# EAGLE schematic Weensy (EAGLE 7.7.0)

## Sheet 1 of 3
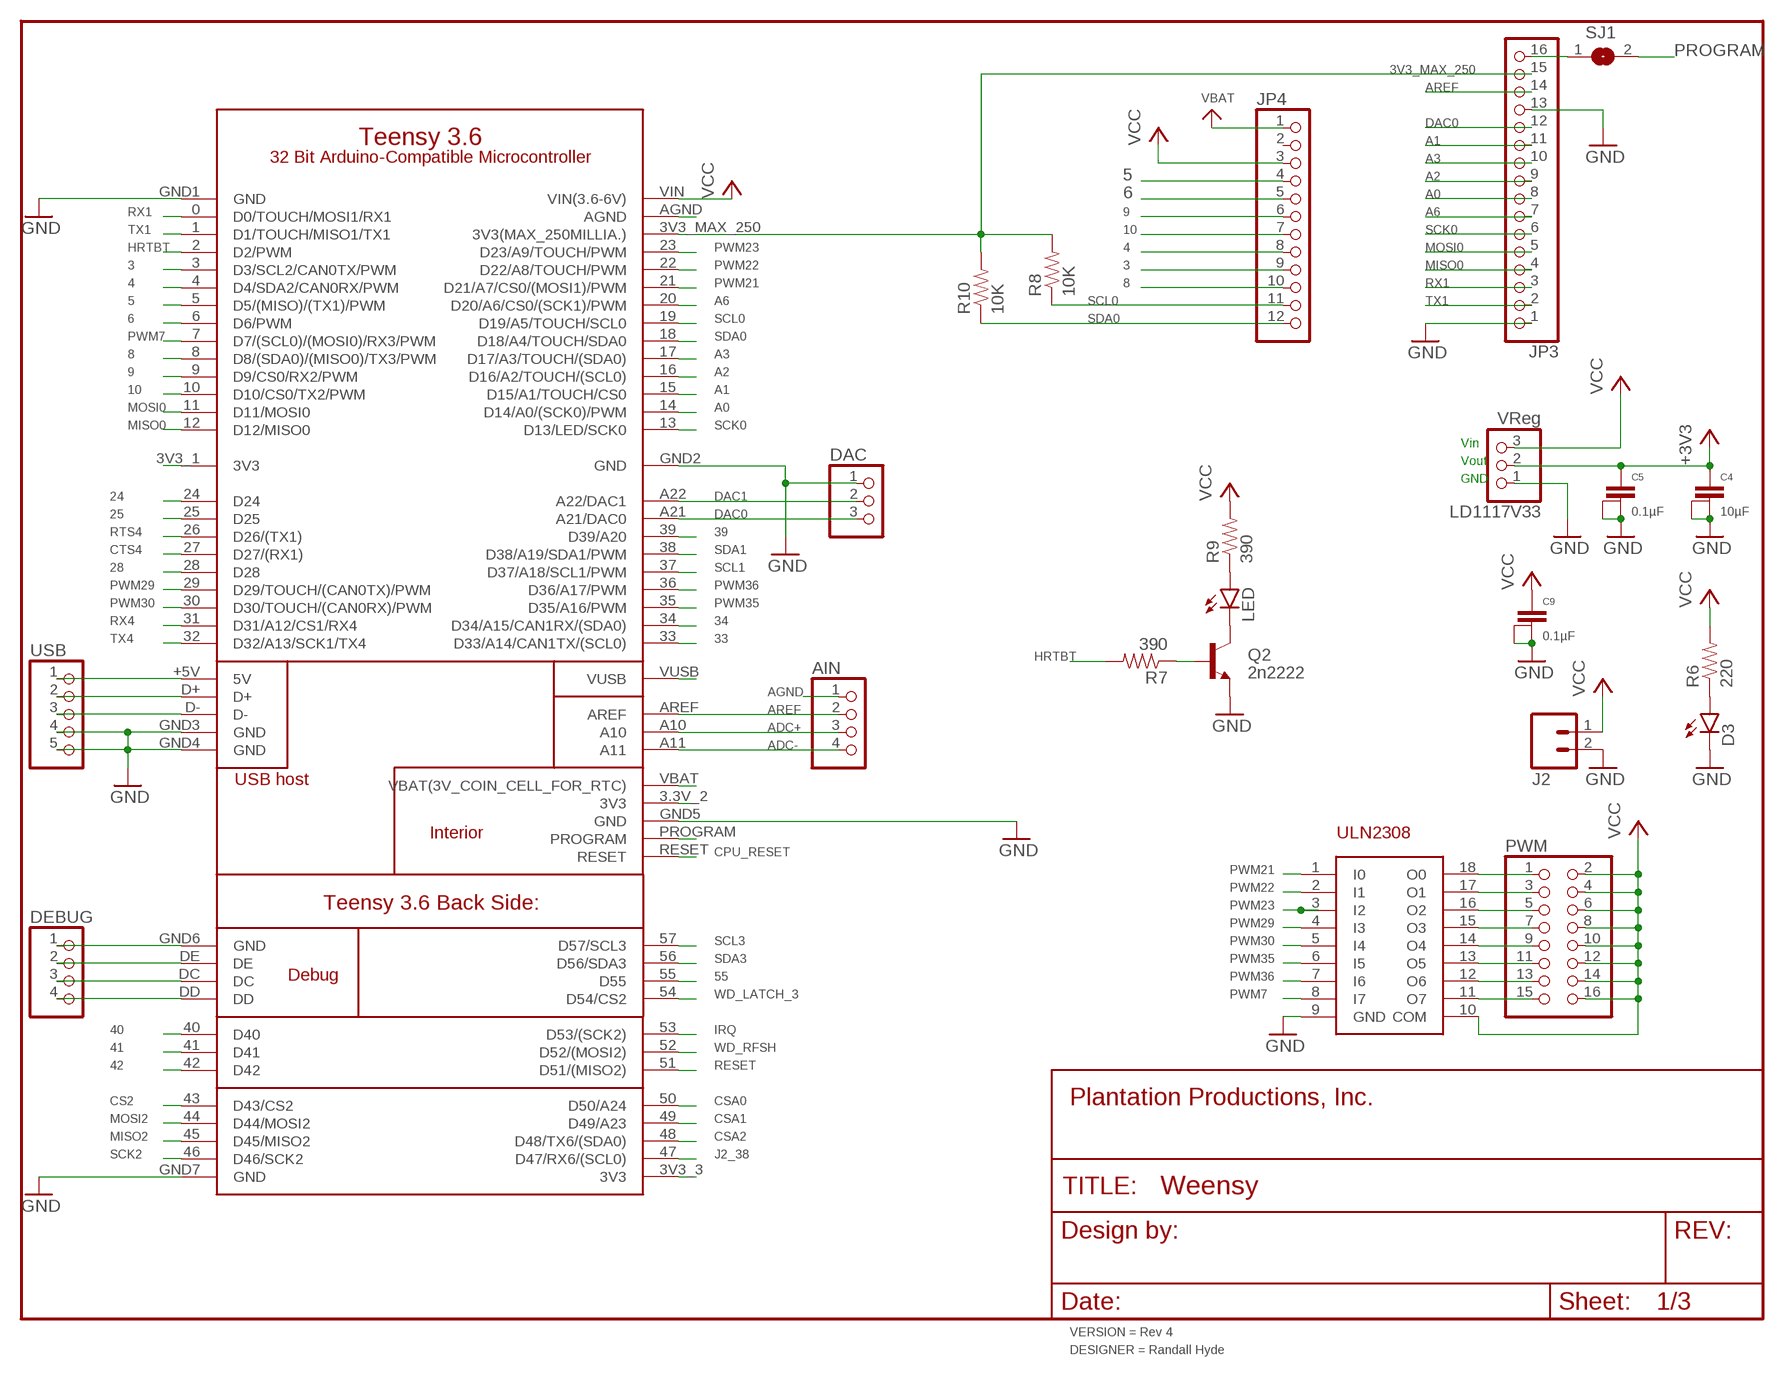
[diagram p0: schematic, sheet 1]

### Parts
AIN  PINHD-1X4  [1X04]
C4  10µF  CAPACITOR  [1+2CAP]
C5  0.1µF  CAPACITOR  [1+2CAP]
C9  0.1µF  CAPACITOR  [1+2CAP]
D3  LED5MM  [LED5MM]
DAC  PINHD-1X3  [1X03]
DEBUG  PINHD-1X4  [1X04]
FRAME1  FRAME-LETTERNO_PACKAGE  [DUMMY]
J2  M025MM  [SCREWTERMINAL-5MM-2]
JP3  HEADER-1X16ROUND  [1X16_ROUND]
JP4  HEADER-1X12  [1X12_ROUND]
LD1117V33  VReg  PINHD-1X3  [1X03]
LED  LED5MM  [LED5MM]
PWM  PINHD-2X8  [2X08]
Q2  2n2222  TRANSISTOR_NPNP2N2222A  [TO-92]
R6  220  1KOHM-1/4W-1%(PTH)  [AXIAL-0.3]
R7  390  10KOHM-1/4W-1%(PTH)HORIZ  [AXIAL-0.3]
R8  10K  10KOHM-1/4W-1%(PTH)HORIZ  [AXIAL-0.3]
R9  390  10KOHM-1/4W-1%(PTH)HORIZ  [AXIAL-0.3]
R10  10K  10KOHM-1/4W-1%(PTH)HORIZ  [AXIAL-0.3]
SJ1  SOLDERJUMPERCLOSED  [SOLDERJUMPER_CLOSEDWIRE]
U$1  TEENSY-3.6_FULL  [TEENSY-3.6_FULL]
ULN2308  ULN2308  [DIL18]
USB  PINHD-1X5  [1X05]

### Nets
3: JP4.9 U$1.3(D3/SCL2/CAN0TX/PWM)
3V3_MAX_250: JP3.15 R8.P$2 R10.P$2 U$1.3V3_MAX_250(3V3(MAX_250MILLIA.))
4: JP4.8 U$1.4(D4/SDA2/CAN0RX/PWM)
5: JP4.4 U$1.5(D5/(MISO)/(TX1)/PWM)
6: JP4.5 U$1.6(D6/PWM)
8: JP4.10 U$1.8(D8/(SDA0)/(MISO0)/TX3/PWM)
9: JP4.6 U$1.9(D9/CS0/RX2/PWM)
10: JP4.7 U$1.10(D10/CS0/TX2/PWM)
24: U$1.24(D24) ; also sheet 2
25: U$1.25(D25) ; also sheet 2
28: U$1.28(D28) ; also sheet 2
33: U$1.33(D33/A14/CAN1TX/(SCL0)) ; also sheet 2
34: U$1.34(D34/A15/CAN1RX/(SDA0)) ; also sheet 2
39: U$1.39(D39/A20) ; also sheet 2
40: U$1.40(D40) ; also sheet 2
41: U$1.41(D41) ; also sheet 2
42: U$1.42(D42) ; also sheet 2
55: U$1.55(D55) ; also sheet 2
+3V3 [Power]: C4.1 C5.1 LD1117V33.2 ; also sheet 2,3
A0: JP3.8 U$1.14(D14/A0/(SCK0)/PWM)
A1: JP3.11 U$1.15(D15/A1/TOUCH/CS0)
A2: JP3.9 U$1.16(D16/A2/TOUCH/(SCL0))
A3: JP3.10 U$1.17(D17/A3/TOUCH/(SDA0))
A6: JP3.7 U$1.20(D20/A6/CS0/(SCK1)/PWM)
ADC+: AIN.3 U$1.A10
ADC-: AIN.4 U$1.A11
AGND: AIN.1 U$1.AGND
AREF: AIN.2 JP3.14 U$1.AREF
CPU_RESET: U$1.RESET
CS2: U$1.43(D43/CS2) ; also sheet 3
CSA0: U$1.50(D50/A24) ; also sheet 3
CSA1: U$1.49(D49/A23) ; also sheet 3
CSA2: U$1.48(D48/TX6/(SDA0)) ; also sheet 3
CTS4: U$1.27(D27/(RX1)) ; also sheet 3
DAC0: DAC.3 JP3.12 U$1.A21(A21/DAC0)
DAC1: DAC.2 U$1.A22(A22/DAC1)
GND: C4.2@1 C4.2@2 C5.2@1 C5.2@2 C9.2@1 C9.2@2 D3.K(C) DAC.1 DEBUG.1 J2.2 JP3.1 JP3.13 LD1117V33.1 Q2.3(E) U$1.GND1(GND) U$1.GND2(GND) U$1.GND3(GND) U$1.GND4(GND) U$1.GND5(GND) U$1.GND6(GND) U$1.GND7(GND) ULN2308.9(GND) USB.4 USB.5 ; also sheet 2,3
HRTBT: R7.P$2 U$1.2(D2/PWM)
IRQ: U$1.53(D53/(SCK2)) ; also sheet 2
J2_38: U$1.47(D47/RX6/(SCL0)) ; also sheet 2
MISO0: JP3.4 U$1.12(D12/MISO0)
MISO2: U$1.45(D45/MISO2) ; also sheet 2
MOSI0: JP3.5 U$1.11(D11/MOSI0)
MOSI2: U$1.44(D44/MOSI2) ; also sheet 2
N$2: D3.A R6.P$1
N$20 [Power]: U$1.3V3_3(3V3)
N$23 [Hi Current]: PWM.1 ULN2308.18(O0)
N$24 [Hi Current]: PWM.3 ULN2308.17(O1)
N$25 [Hi Current]: PWM.5 ULN2308.16(O2)
N$26 [Hi Current]: PWM.7 ULN2308.15(O3)
N$27 [Hi Current]: PWM.9 ULN2308.14(O4)
N$28 [Hi Current]: PWM.11 ULN2308.13(O5)
N$29 [Hi Current]: PWM.13 ULN2308.12(O6)
N$30 [Hi Current]: PWM.15 ULN2308.11(O7)
N$31: U$1.3V3_1(3V3)
N$36: LED.K(C) Q2.1(C)
N$37: Q2.2(B) R7.P$1
N$38: LED.A R9.P$1
N$41: U$1.+5V(5V) USB.1
N$42: U$1.D+ USB.2
N$43: U$1.D- USB.3
N$46: DEBUG.2 U$1.DE
N$47: DEBUG.3 U$1.DC
N$48: DEBUG.4 U$1.DD
N$71: U$1.3.3V_2(3V3)
PROGRAM: SJ1.2 U$1.PROGRAM
PWM7: U$1.7(D7/(SCL0)/(MOSI0)/RX3/PWM) ULN2308.8(I7)
PWM21: U$1.21(D21/A7/CS0/(MOSI1)/PWM) ULN2308.1(I0)
PWM22: U$1.22(D22/A8/TOUCH/PWM) ULN2308.2(I1)
PWM23: U$1.23(D23/A9/TOUCH/PWM) ULN2308.3(I2)
PWM29: U$1.29(D29/TOUCH/(CAN0TX)/PWM) ULN2308.4(I3)
PWM30: U$1.30(D30/TOUCH/(CAN0RX)/PWM) ULN2308.5(I4)
PWM35: U$1.35(D35/A16/PWM) ULN2308.6(I5)
PWM36: U$1.36(D36/A17/PWM) ULN2308.7(I6)
RESET: U$1.51(D51/(MISO2)) ; also sheet 2,3
RST/BOOT: JP3.16 SJ1.1
RTS4: U$1.26(D26/(TX1)) ; also sheet 3
RX1: JP3.3 U$1.0(D0/TOUCH/MOSI1/RX1)
RX4: U$1.31(D31/A12/CS1/RX4) ; also sheet 3
SCK0: JP3.6 U$1.13(D13/LED/SCK0)
SCK2: U$1.46(D46/SCK2) ; also sheet 2,3
SCL0: JP4.11 R8.P$1 U$1.19(D19/A5/TOUCH/SCL0)
SCL1: U$1.37(D37/A18/SCL1/PWM) ; also sheet 2
SCL3: U$1.57(D57/SCL3) ; also sheet 2
SDA0: JP4.12 R10.P$1 U$1.18(D18/A4/TOUCH/SDA0)
SDA1: U$1.38(D38/A19/SDA1/PWM) ; also sheet 2
SDA3: U$1.56(D56/SDA3) ; also sheet 2
TX1: JP3.2 U$1.1(D1/TOUCH/MISO1/TX1)
TX4: U$1.32(D32/A13/SCK1/TX4) ; also sheet 3
VBAT: JP4.1 U$1.VBAT(VBAT(3V_COIN_CELL_FOR_RTC))
VCC [Hi Current]: C9.1 J2.1 JP4.3 LD1117V33.3 PWM.2 PWM.4 PWM.6 PWM.8 PWM.10 PWM.12 PWM.14 PWM.16 R6.P$2 R9.P$2 U$1.VIN(VIN(3.6-6V)) ULN2308.10(COM) ; also sheet 2,3
VUSB: U$1.VUSB
WD_LATCH_3: U$1.54(D54/CS2) ; also sheet 2
WD_RFSH: U$1.52(D52/(MOSI2)) ; also sheet 2
Unconnected: JP4.2

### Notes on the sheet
- Vin
- Vout
- GND

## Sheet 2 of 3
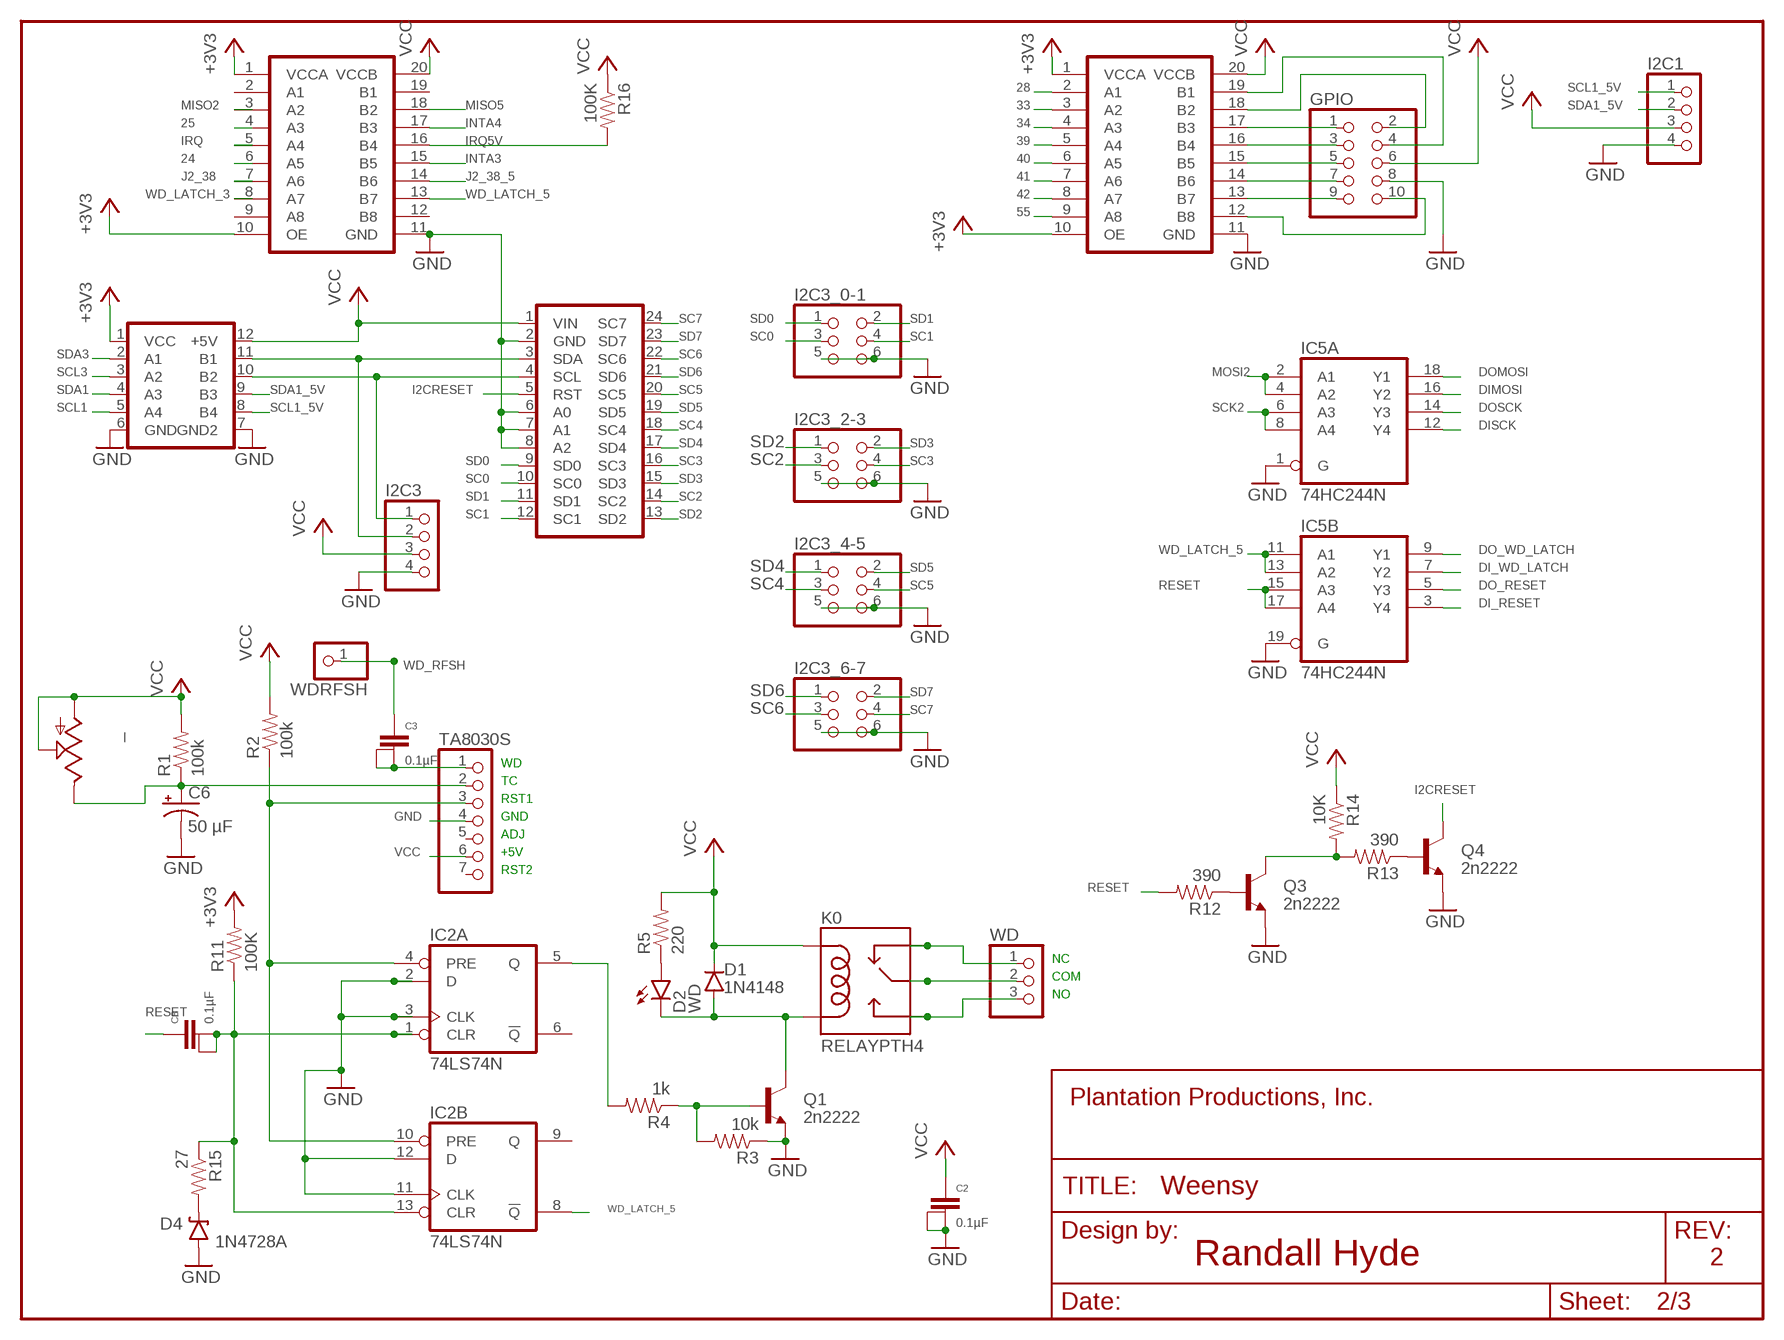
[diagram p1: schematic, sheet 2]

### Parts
_  TRIM_US-B64Y  [B64Y]
BOB1  ADAFRTTXB0108  [DIL20W]
BOB2  ADAFRTBSS138  [DIL12W]
BOB3  ADAFRTTCA9584  [DIL24W]
BOB4  ADAFRTTXB0108  [DIL20W]
C2  0.1µF  CAPACITOR  [1+2CAP]
C3  0.1µF  CAPACITOR  [1+2CAP]
C6  50 µF  100UF-25V-20%(PTH)  [CPOL-RADIAL-100UF-25V]
C8  0.1µF  CAPACITOR  [1+2CAP]
D1  1N4148  DIODE1N4148  [DIODE-1N4148]
D2  WD  LED5MM  [LED5MM]
D4  1N4728A  DIODE-ZENERPTH  [DIODE-ZENER]
FRAME2  FRAME-LETTERNO_PACKAGE  [DUMMY]
GPIO  PINHD-2X5  [2X05]
I2C1  PINHD-1X4  [1X04]
I2C3  PINHD-1X4  [1X04]
I2C3_0-1  PINHD-2X3  [2X03]
I2C3_2-3  PINHD-2X3  [2X03]
I2C3_4-5  PINHD-2X3  [2X03]
I2C3_6-7  PINHD-2X3  [2X03]
IC2  74LS74N  [DIL14]
IC5  74HC244N  [DIL20]
K0  RELAYPTH4  [RELAY-JZC]
Q1  2n2222  TRANSISTOR_NPNP2N2222A  [TO-92]
Q3  2n2222  TRANSISTOR_NPNP2N2222A  [TO-92]
Q4  2n2222  TRANSISTOR_NPNP2N2222A  [TO-92]
R1  100k  10KOHM-1/4W-1%(PTH)HORIZ  [AXIAL-0.3]
R2  100k  10KOHM-1/4W-1%(PTH)HORIZ  [AXIAL-0.3]
R3  10k  10KOHM-1/4W-1%(PTH)HORIZ  [AXIAL-0.3]
R4  1k  10KOHM-1/4W-1%(PTH)HORIZ  [AXIAL-0.3]
R5  220  10KOHM-1/4W-1%(PTH)HORIZ  [AXIAL-0.3]
R11  100K  1KOHM-1/4W-1%(PTH)  [AXIAL-0.3]
R12  390  10KOHM-1/4W-1%(PTH)HORIZ  [AXIAL-0.3]
R13  390  10KOHM-1/4W-1%(PTH)HORIZ  [AXIAL-0.3]
R14  10K  10KOHM-1/4W-1%(PTH)HORIZ  [AXIAL-0.3]
R15  27  1KOHM-1/4W-1%(PTH)  [AXIAL-0.3]
R16  100K  10KOHM-1/4W-1%(PTH)HORIZ  [AXIAL-0.3]
TA8030S  PINHD-1X7  [1X07]
WD  PINHD-1X3  [1X03]
WDRFSH  PINHD-1X1  [1X01]

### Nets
24: BOB1.6(A5) ; also sheet 1
25: BOB1.4(A3) ; also sheet 1
28: BOB4.2(A1) ; also sheet 1
33: BOB4.3(A2) ; also sheet 1
34: BOB4.4(A3) ; also sheet 1
39: BOB4.5(A4) ; also sheet 1
40: BOB4.6(A5) ; also sheet 1
41: BOB4.7(A6) ; also sheet 1
42: BOB4.8(A7) ; also sheet 1
55: BOB4.9(A8) ; also sheet 1
+3V3 [Power]: BOB1.1(VCCA) BOB1.10(OE) BOB2.1(VCC) BOB4.1(VCCA) BOB4.10(OE) R11.P$2 ; also sheet 1,3
DI_RESET: IC5.3(B:Y4) ; also sheet 3
DI_WD_LATCH: IC5.7(B:Y2) ; also sheet 3
DIMOSI: IC5.16(A:Y2) ; also sheet 3
DISCK: IC5.12(A:Y4) ; also sheet 3
DO_RESET: IC5.5(B:Y3) ; also sheet 3
DO_WD_LATCH: IC5.9(B:Y1) ; also sheet 3
DOMOSI: IC5.18(A:Y1) ; also sheet 3
DOSCK: IC5.14(A:Y3) ; also sheet 3
GND: BOB1.11(GND) BOB2.6(GND) BOB2.7(GND2) BOB3.2(GND) BOB3.6(A0) BOB3.7(A1) BOB3.8(A2) BOB4.11(GND) C2.2@1 C2.2@2 C6.2(-) D4.P$2(A) GPIO.8 I2C1.4 I2C3.4 I2C3_0-1.5 I2C3_0-1.6 I2C3_2-3.5 I2C3_2-3.6 I2C3_4-5.5 I2C3_4-5.6 I2C3_6-7.5 I2C3_6-7.6 IC2.2(A:D) IC2.3(A:CLK) IC2.11(B:CLK) IC2.12(B:D) IC5.1(A:G) IC5.19(B:G) Q1.3(E) Q3.3(E) Q4.3(E) R3.P$1 TA8030S.4 ; also sheet 1,3
GPIO28: BOB4.19(B1) GPIO.4
GPIO33: BOB4.18(B2) GPIO.2
GPIO34: BOB4.17(B3) GPIO.1
GPIO39: BOB4.16(B4) GPIO.3
GPIO40: BOB4.15(B5) GPIO.5
GPIO41: BOB4.14(B6) GPIO.7
GPIO42: BOB4.13(B7) GPIO.9
GPIO55: BOB4.12(B8) GPIO.10
I2CRESET: BOB3.5(RST) Q4.1(C)
INTA3: BOB1.15(B5) ; also sheet 3
INTA4: BOB1.17(B3) ; also sheet 3
IRQ: BOB1.5(A4) ; also sheet 1
IRQ5V: BOB1.16(B4) R16.P$2 ; also sheet 3
J2_38: BOB1.7(A6) ; also sheet 1
J2_38_5: BOB1.14(B6) ; also sheet 3
MISO2: BOB1.3(A2) ; also sheet 1
MISO5: BOB1.18(B2) ; also sheet 3
MOSI2: IC5.2(A:A1) IC5.4(A:A2) ; also sheet 1
N$3: C3.2@1 C3.2@2 TA8030S.1
N$4: _.E C6.1(+) R1.P$1 TA8030S.2
N$5: BOB2.11(B1) BOB3.3(SDA) I2C3.2
N$6: D1.A D2.K(C) K0.1(COIL2) Q1.1(C)
N$9: D2.A R5.P$1
N$11: Q1.2(B) R3.P$2 R4.P$1
N$12: Q3.2(B) R12.P$1
N$13: Q4.2(B) R13.P$1
N$14 [Power]: K0.4(MAIN) WD.2
N$15 [Power]: K0.3(NO) WD.3
N$16: BOB2.10(B2) BOB3.4(SCL) I2C3.1
N$17: Q3.1(C) R13.P$2 R14.P$2
N$39: D4.P$1(C) R15.P$2
NC [Power]: K0.2(NC) WD.1
RESET: C8.1 IC5.15(B:A3) IC5.17(B:A4) R12.P$2 ; also sheet 1,3
RESETWD: C8.2@1 C8.2@2 IC2.1(A:CLR) IC2.13(B:CLR) R11.P$1 R15.P$1
RST1: IC2.4(A:PRE) IC2.10(B:PRE) R2.P$1 TA8030S.3
SC0: BOB3.10(SC0) I2C3_0-1.3
SC1: BOB3.12(SC1) I2C3_0-1.4
SC2: BOB3.14(SC2) I2C3_2-3.3
SC3: BOB3.16(SC3) I2C3_2-3.4
SC4: BOB3.18(SC4) I2C3_4-5.3
SC5: BOB3.20(SC5) I2C3_4-5.4
SC6: BOB3.22(SC6) I2C3_6-7.3
SC7: BOB3.24(SC7) I2C3_6-7.4
SCK2: IC5.6(A:A3) IC5.8(A:A4) ; also sheet 1,3
SCL1: BOB2.5(A4) ; also sheet 1
SCL1_5V: BOB2.8(B4) I2C1.1
SCL3: BOB2.3(A2) ; also sheet 1
SD0: BOB3.9(SD0) I2C3_0-1.1
SD1: BOB3.11(SD1) I2C3_0-1.2
SD2: BOB3.13(SD2) I2C3_2-3.1
SD3: BOB3.15(SD3) I2C3_2-3.2
SD4: BOB3.17(SD4) I2C3_4-5.1
SD5: BOB3.19(SD5) I2C3_4-5.2
SD6: BOB3.21(SD6) I2C3_6-7.1
SD7: BOB3.23(SD7) I2C3_6-7.2
SDA1: BOB2.4(A3) ; also sheet 1
SDA1_5V: BOB2.9(B3) I2C1.2
SDA3: BOB2.2(A1) ; also sheet 1
VCC [Hi Current]: _.A _.S BOB1.20(VCCB) BOB2.12(+5V) BOB3.1(VIN) BOB4.20(VCCB) C2.1 D1.C GPIO.6 I2C1.3 I2C3.3 K0.5(COIL1) R1.P$2 R2.P$2 R5.P$2 R14.P$1 R16.P$1 TA8030S.6 ; also sheet 1,3
WD_LATCH_3: BOB1.8(A7) ; also sheet 1
WD_LATCH_5: BOB1.13(B7) IC2.8(B:!Q) IC5.11(B:A1) IC5.13(B:A2)
WD_RFSH: C3.1 WDRFSH.1 ; also sheet 1
WDOUT: IC2.5(A:Q) R4.P$2
Unconnected: BOB1.2(A1) BOB1.9(A8) BOB1.12(B8) BOB1.19(B1) IC2.6(A:!Q) IC2.9(B:Q) TA8030S.5 TA8030S.7

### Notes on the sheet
- WD
- TC
- RST1
- GND
- ADJ
- +5V
- RST2
- NC
- COM
- NO
- Randall Hyde | 2

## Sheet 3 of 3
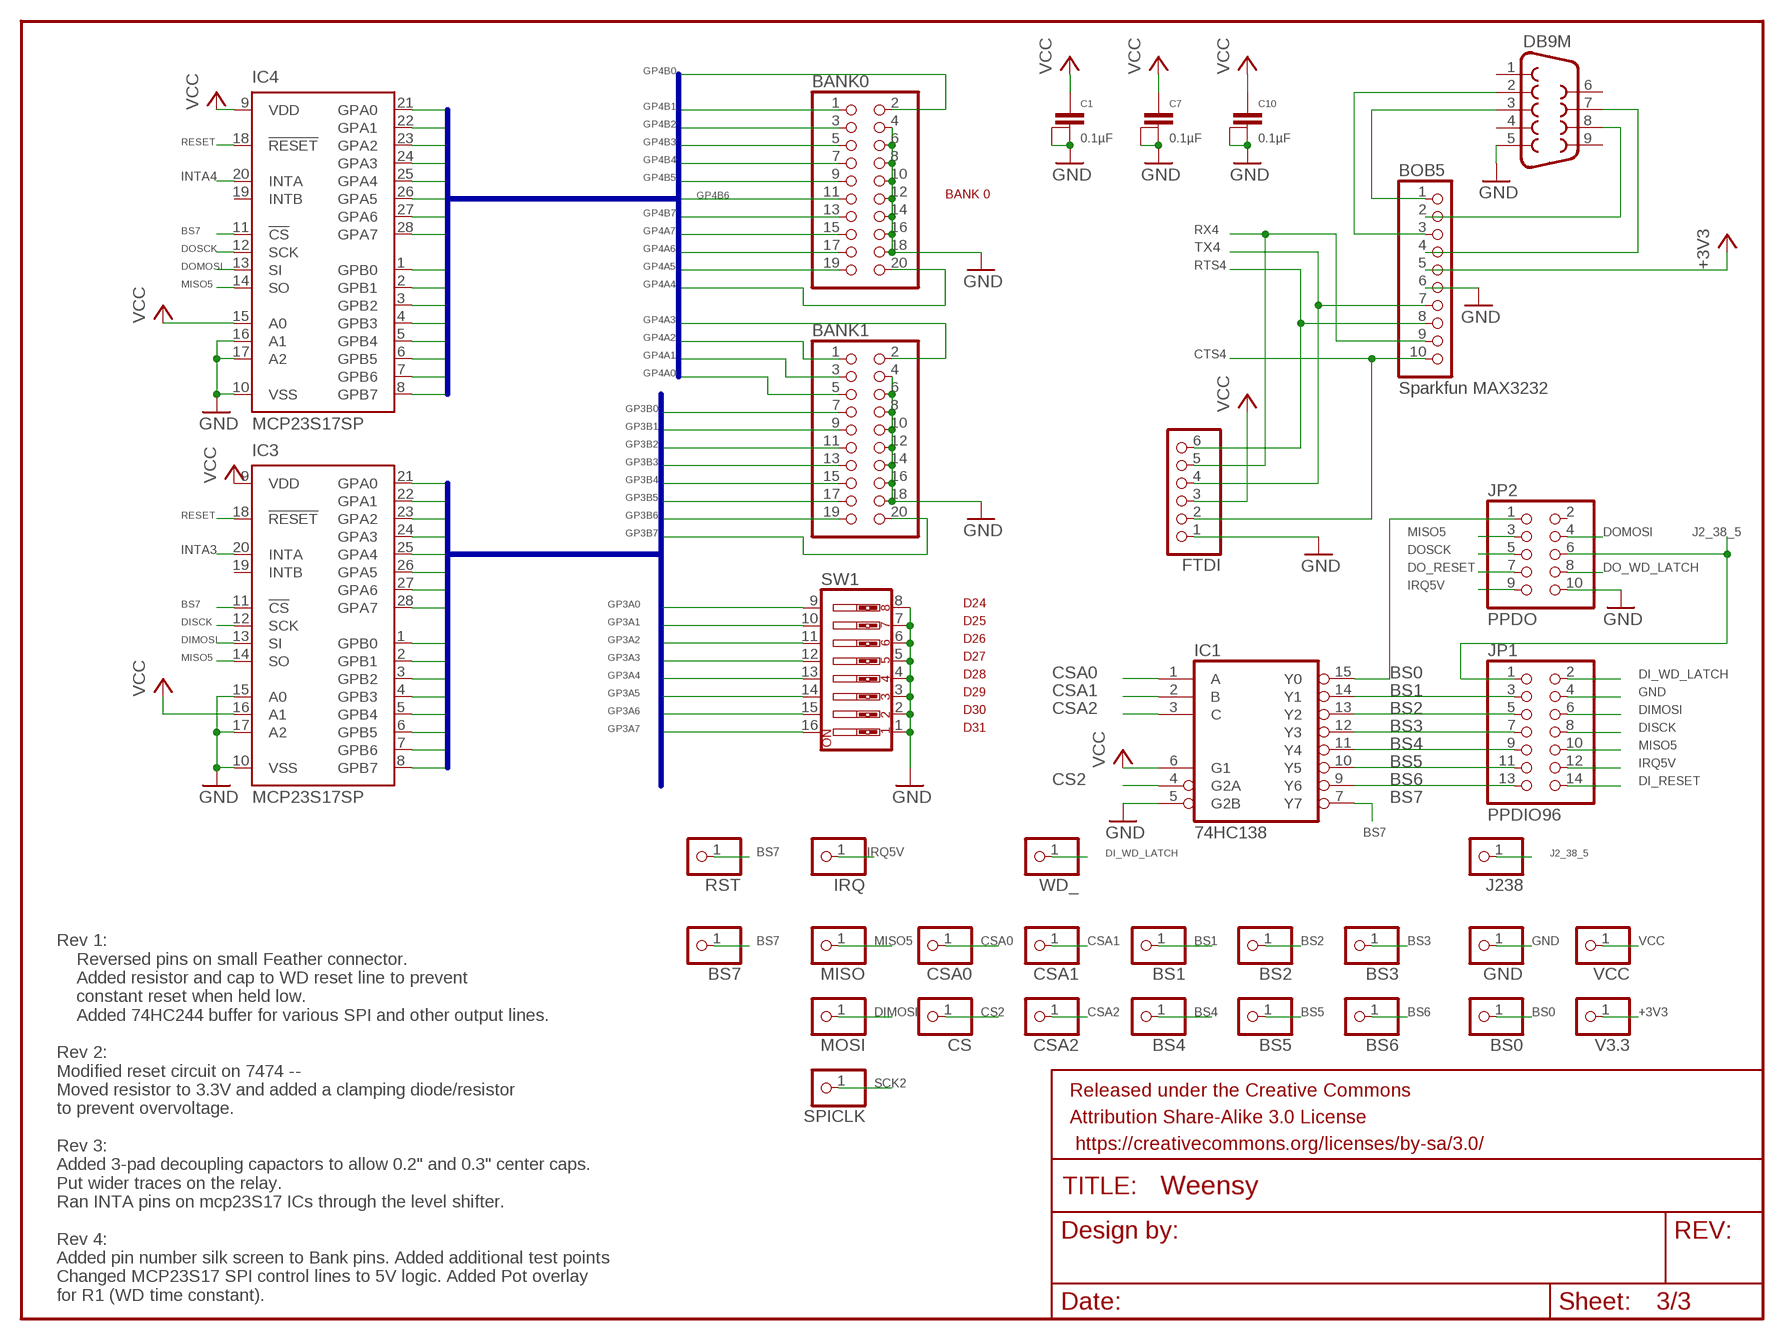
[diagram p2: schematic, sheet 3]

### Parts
BANK0  PINHD-2X10  [2X10]
BANK1  PINHD-2X10  [2X10]
BOB5  Sparkfun MAX3232  PINHD-1X10  [1X10]
BS0  PINHD-1X1  [1X01]
BS1  PINHD-1X1  [1X01]
BS2  PINHD-1X1  [1X01]
BS3  PINHD-1X1  [1X01]
BS4  PINHD-1X1  [1X01]
BS5  PINHD-1X1  [1X01]
BS6  PINHD-1X1  [1X01]
BS7  PINHD-1X1  [1X01]
C1  0.1µF  CAPACITOR  [1+2CAP]
C7  0.1µF  CAPACITOR  [1+2CAP]
C10  0.1µF  CAPACITOR  [1+2CAP]
CS  PINHD-1X1  [1X01]
CSA0  PINHD-1X1  [1X01]
CSA1  PINHD-1X1  [1X01]
CSA2  PINHD-1X1  [1X01]
DB9M  DB9MALE  [DB9_MALE]
FRAME3  FRAME-LETTER  [CREATIVE_COMMONS]
FTDI  PINHD-1X6  [1X06]
GND  PINHD-1X1  [1X01]
IC1  74HC138  74LS138N  [DIL16]
IC3  MCP23S17SP  [DIL28-3]
IC4  MCP23S17SP  [DIL28-3]
IRQ  PINHD-1X1  [1X01]
J238  PINHD-1X1  [1X01]
JP1  PPDIO96  PINHD-2X7  [2X07]
JP2  PPDO  PINHD-2X5  [2X05]
MISO  PINHD-1X1  [1X01]
MOSI  PINHD-1X1  [1X01]
RST  PINHD-1X1  [1X01]
SPICLK  PINHD-1X1  [1X01]
SW1  SW_DIP-8  [DIPSWITCH-08]
V3.3  PINHD-1X1  [1X01]
VCC  PINHD-1X1  [1X01]
WD_  PINHD-1X1  [1X01]

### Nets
+3V3 [Power]: BOB5.5 V3.3.1 ; also sheet 1,2
BS0: BS0.1 IC1.15(Y0) JP2.1
BS1: BS1.1 IC1.14(Y1) JP1.3
BS2: BS2.1 IC1.13(Y2) JP1.5
BS3: BS3.1 IC1.12(Y3) JP1.7
BS4: BS4.1 IC1.11(Y4) JP1.9
BS5: BS5.1 IC1.10(Y5) JP1.11
BS6: BS6.1 IC1.9(Y6) JP1.13
BS7: BS7.1 IC1.7(Y7) IC3.11(!CS) IC4.11(!CS) RST.1
CS2: CS.1 IC1.4(G2A) ; also sheet 1
CSA0: CSA0.1 IC1.1(A) ; also sheet 1
CSA1: CSA1.1 IC1.2(B) ; also sheet 1
CSA2: CSA2.1 IC1.3(C) ; also sheet 1
CTS4: BOB5.10 FTDI.2 ; also sheet 1
DI_RESET: JP1.14 ; also sheet 2
DI_WD_LATCH: JP1.2 WD_.1 ; also sheet 2
DIMOSI: IC3.13(SI) JP1.6 MOSI.1 ; also sheet 2
DISCK: IC3.12(SCK) JP1.8 ; also sheet 2
DO_RESET: JP2.7 ; also sheet 2
DO_WD_LATCH: JP2.8 ; also sheet 2
DOMOSI: IC4.13(SI) JP2.4 ; also sheet 2
DOSCK: IC4.12(SCK) JP2.5 ; also sheet 2
GND: BANK0.4 BANK0.6 BANK0.8 BANK0.10 BANK0.12 BANK0.14 BANK0.16 BANK0.18 BANK1.4 BANK1.6 BANK1.8 BANK1.10 BANK1.12 BANK1.14 BANK1.16 BANK1.18 BOB5.6 C1.2@1 C1.2@2 C7.2@1 C7.2@2 C10.2@1 C10.2@2 DB9M.5 FTDI.1 GND.1 IC1.5(G2B) IC3.10(VSS) IC3.15(A0) IC3.17(A2) IC4.10(VSS) IC4.16(A1) IC4.17(A2) JP1.4 JP2.10 SW1.1 SW1.2 SW1.3 SW1.4 SW1.5 SW1.6 SW1.7 SW1.8 ; also sheet 1,2
GP3A0: IC3.28(GPA7) SW1.9
GP3A1: IC3.27(GPA6) SW1.10
GP3A2: IC3.26(GPA5) SW1.11
GP3A3: IC3.25(GPA4) SW1.12
GP3A4: IC3.24(GPA3) SW1.13
GP3A5: IC3.23(GPA2) SW1.14
GP3A6: IC3.22(GPA1) SW1.15
GP3A7: IC3.21(GPA0) SW1.16
GP3B0: BANK1.7 IC3.1(GPB0)
GP3B1: BANK1.9 IC3.2(GPB1)
GP3B2: BANK1.11 IC3.3(GPB2)
GP3B3: BANK1.13 IC3.4(GPB3)
GP3B4: BANK1.15 IC3.5(GPB4)
GP3B5: BANK1.17 IC3.6(GPB5)
GP3B6: BANK1.19 IC3.7(GPB6)
GP3B7: BANK1.20 IC3.8(GPB7)
GP4A0: BANK1.5 IC4.21(GPA0)
GP4A1: BANK1.3 IC4.22(GPA1)
GP4A2: BANK1.1 IC4.23(GPA2)
GP4A3: BANK1.2 IC4.24(GPA3)
GP4A4: BANK0.20 IC4.25(GPA4)
GP4A5: BANK0.19 IC4.26(GPA5)
GP4A6: BANK0.17 IC4.27(GPA6)
GP4A7: BANK0.15 IC4.28(GPA7)
GP4B0: BANK0.2 IC4.1(GPB0)
GP4B1: BANK0.1 IC4.2(GPB1)
GP4B2: BANK0.3 IC4.3(GPB2)
GP4B3: BANK0.5 IC4.4(GPB3)
GP4B4: BANK0.7 IC4.5(GPB4)
GP4B5: BANK0.9 IC4.6(GPB5)
GP4B6: BANK0.11 IC4.7(GPB6)
GP4B7: BANK0.13 IC4.8(GPB7)
INTA3: IC3.20(INTA) ; also sheet 2
INTA4: IC4.20(INTA) ; also sheet 2
IRQ5V: IRQ.1 JP1.12 JP2.9 ; also sheet 2
J2_38_5: J238.1 JP1.1 JP2.6 ; also sheet 2
MISO5: IC3.14(SO) IC4.14(SO) JP1.10 JP2.3 MISO.1 ; also sheet 2
N$32: BOB5.2 DB9M.8
N$33: BOB5.4 DB9M.7
N$34: BOB5.1 DB9M.3
N$35: BOB5.3 DB9M.2
RESET: IC3.18(!RESET) IC4.18(!RESET) ; also sheet 1,2
RTS4: BOB5.8 FTDI.6 ; also sheet 1
RX4: BOB5.9 FTDI.5 ; also sheet 1
SCK2: SPICLK.1 ; also sheet 1,2
TX4: BOB5.7 FTDI.4 ; also sheet 1
VCC [Hi Current]: C1.1 C7.1 C10.1 FTDI.3 IC1.6(G1) IC3.9(VDD) IC3.16(A1) IC4.9(VDD) IC4.15(A0) VCC.1 ; also sheet 1,2
Unconnected: DB9M.1 DB9M.4 DB9M.6 DB9M.9 IC3.19(INTB) IC4.19(INTB) JP2.2

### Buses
IC2BUS:GP4A[0..7],GP4B[0..7]
IC3BUS:GP3A[0..7],GP3B[0..7]

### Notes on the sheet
- BANK 0
- D24
- D25
- D26
- D27
- D28
- D29
- D30
- D31
- Rev 1:
      Reversed pins on small Feather connector.
      Added resistor and cap to WD reset line to prevent
      constant reset when held low.
      Added 74HC244 buffer for various SPI and other output lines.
  
  Rev 2:
  Modified reset circuit on 7474 -- 
  Moved resistor to 3.3V and added a clamping diode/resistor 
  to prevent overvoltage.
  
  Rev 3:
  Added 3-pad decoupling capactors to allow 0.2" and 0.3" center caps.
  Put wider traces on the relay.
  Ran INTA pins on mcp23S17 ICs through the level shifter.
  
  Rev 4:
  Added pin number silk screen to Bank pins. Added additional test points
  Changed MCP23S17 SPI control lines to 5V logic. Added Pot overlay
  for R1 (WD time constant).

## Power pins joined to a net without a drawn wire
GND: IC1.8(GND) IC2.7(P:GND) IC5.10(P:GND)
VCC: IC1.16(VCC) IC2.14(P:VCC) IC5.20(P:VCC)

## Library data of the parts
_ = pot:TRIM_US-: POTENTIOMETER
AIN DEBUG I2C1 I2C3 = pinhead:PINHD-1X4: PIN HEADER
BANK0 BANK1 = SparkFun-Connectors:PINHD-2X10: PIN HEADER
BOB1 BOB4 = PlantProd:ADAFRTTXB0108: AdaFruit TXB0108 8-channel level shifter
BOB2 = PlantProd:ADAFRTBSS138: AdaFruit BSS138 4-channel I2C bi-directional logical level converter
BOB3 = PlantProd:ADAFRTTCA9584: AdaFruit TCA9548A 8-channel I2C multiplexer
BOB5 = pinhead:PINHD-1X10: PIN HEADER
BS0 BS1-BS7 CS CSA0 CSA1 CSA2 GND IRQ J238 MISO MOSI RST SPICLK V3.3 VCC WD_ WDRFSH = pinhead:PINHD-1X1: PIN HEADER
C1-C5 C7-C10 = PlantProd:CAPACITOR: Capacitor with three terminals to support multiple capacitor sizes.
C6 = SparkFun-Capacitors:100UF-25V-20%(PTH): CAP-08439; PROD_ID: CAP-08439
D1 = SparkFun-DiscreteSemi:DIODE: Diode; PROD_ID: DIO-08378
D2 D3 LED = SparkFun-LED:LED: LEDs
D4 = SparkFun-DiscreteSemi:DIODE-ZENER: Zener Diode
DAC LD1117V33 WD = pinhead:PINHD-1X3: PIN HEADER
DB9M = SparkFun-Connectors:DB9: DB9 Connector Standard DB9 (D-Sub 9) serial connector. Can be used for CAN bus as well as RS485 and RS232. Footprint production proven. Spark Fun Electronics SKU : PRT-00429; PROD_ID: CONN-09904
FRAME1 = SparkFun-Aesthetics:FRAME-LETTER: Schematic Frame; DESIGNER: Randall Hyde; VERSION: Rev 4
FRAME2 = SparkFun-Aesthetics:FRAME-LETTER: Schematic Frame; DESIGNER: Nobody; VERSION: v01
FRAME3 = SparkFun-Retired:FRAME-LETTER: Schematic Frame
FTDI = pinhead:PINHD-1X6: PIN HEADER
GPIO JP2 = pinhead:PINHD-2X5: PIN HEADER
I2C3_0-1 I2C3_2-3 I2C3_4-5 I2C3_6-7 = pinhead:PINHD-2X3: PIN HEADER
IC1 = 74xx-us:74*138: 3-line to 8-line DECODER/DEMULTIPLEXER
IC2 = 74xx-us:74*74: Dual D type positive edge triggered FLIP FLOP, preset and clear
IC3 IC4 = microchip:MCP23S17: http://ww1.microchip.com/downloads/en/DeviceDoc/21952a.pdf Source: http://ww1.microchip.com/downloads/en/DeviceDoc/21952a.pdf; MF: MICROCHIP; MPN: MCP23S17-E/SP; OC_FARNELL: 1292238; OC_NEWARK: 31K2951
IC5 = 74xx-eu:74*244: Octal BUFFER and LINE DRIVER, 3-state
J2 = SparkFun-Connectors:M02: Standard 2-pin 0.1" header. Use with; STOREFRONT_ID: PRT-08432
JP1 = pinhead:PINHD-2X7: PIN HEADER
JP3 = microbuilder:HEADER-1X16: PIN HEADER
JP4 = microbuilder:HEADER-1X12
K0 = SparkFun-Electromechanical:RELAY: SPDT relay (COM-00101)
PWM = pinhead:PINHD-2X8: PIN HEADER
Q1-Q4 = SparkFun-DiscreteSemi:TRANSISTOR_NPN: Generic NPN BJT MMBT2222A - TRANS-08049 (SOT-23, 1A 40V) MPSA42 - TRANS-09116 (SOT-23, 500mA 300V) MMBT5088LT1G - TRANS-11160 (SOT-23, 50 mA 30V) BC547 - COM-08928 (TO-92 45V 100mA) (1.Collector 2.Base 3.Emitter) 2N3904 - COM-00521 (TO-92 40V 200mA) (1.Emitter 2.Base 3.Collector) P2N2222A -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; PROD_ID: TRANS-09536
R1 R2 R4 R5 R7-R10 R12-R14 R16 = SparkFun-Resistors:10KOHM-1/4W-1%(PTH): RES-12183; PROD_ID: RES-12183; VALUE: 10k
R3 = SparkFun-Resistors:10KOHM-1/4W-1%(PTH): RES-12183; PROD_ID: RES-12183
R6 R11 R15 = SparkFun-Resistors:1KOHM-1/4W-1%(PTH): RES-12182; PROD_ID: RES-12182; VALUE: 1K
SJ1 = microbuilder:SOLDERJUMPER: SMD Solder JUMPER
SW1 = SparkFun-Electromechanical:SW_DIP-8: DIP Switch 8 Position
TA8030S = pinhead:PINHD-1X7: PIN HEADER
U$1 = Teensy-3.6:TEENSY-3.6_FULL
ULN2308 = PlantProd:ULN2308: ULN2308 8-Ch Darlington
USB = pinhead:PINHD-1X5: PIN HEADER

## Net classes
1 Power: width 1.016 mm, drill 0.127 mm, clearance 0.254 mm
2 Hi Current: width 0.508 mm, drill 0.254 mm, clearance 0.254 mm
3 Relay: width 2.54 mm, drill 0.254 mm, clearance 0.254 mm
